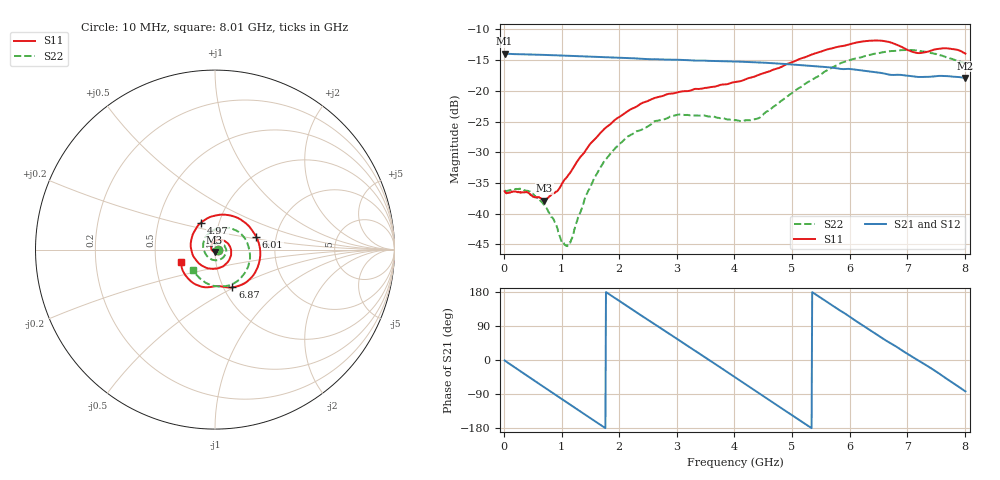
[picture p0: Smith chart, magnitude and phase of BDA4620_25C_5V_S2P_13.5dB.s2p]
!Agilent Technologies,E5071B,MY42404982,A.09.10
!Date: Wed May 06 09:01:02 2026
!Data & Calibration Information:
!Freq	S11:SOLT2(ON)	S21:SOLT2(ON)	S12:SOLT2(ON)	S22:SOLT2(ON)
# Hz S RI R 50
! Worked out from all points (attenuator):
!   801 points, 10 MHz to 8.01 GHz, reference 50 ohm
!   highest |S21| = -13.93 dB at 10 MHz (marker M1); lowest = -17.9 dB at 8.01 GHz (marker M2)
!   lowest |S11| = -37.9 dB at 700 MHz (marker M3), VSWR 1.03, Z = 49.7 - j1.24 ohm
!   |S11| at or under -10 dB: start of sweep to end of sweep
!   |S22| runs from -45.3 to -13.3 dB; largest |S21 - S12| = 0.0009
!   S11 on the Smith chart (normalised r, x): 10 MHz: 1.03, -0.00; 4.97 GHz: 0.82, +0.25; 6.01 GHz: 1.57, +0.24; 6.87 GHz: 1.10, -0.49; 8.01 GHz: 0.68, -0.10
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1e7  0.0152 -0.00103  0.2011 -0.00428  0.2014 -0.00438  0.0154 -0.000666
4.4e8  0.00868 -0.0117  0.1385 -0.1413  0.1386 -0.1417  0.0135 -0.00702
7e8  -0.00256 -0.0125  0.06 -0.1868  0.0599 -0.1872  0.00726 -0.00918
1.08e9  -0.0195 0.00114  -0.0692 -0.1807  -0.0695 -0.181  -0.00435 -0.00332
1.16e9  -0.0208 0.00685  -0.0938 -0.1686  -0.0942 -0.1687  -0.00598 -0.000482
1.35e9  -0.0211 0.0211  -0.1433 -0.1271  -0.1434 -0.1272  -0.00816 0.00748
1.59e9  -0.0112 0.0395  -0.1809 -0.0565  -0.1812 -0.0566  -0.00604 0.0194
1.9e9  0.0164 0.0542  -0.1816 0.0451  -0.1818 0.0452  0.00652 0.0323
2.31e9  0.0618 0.0422  -0.1046 0.1508  -0.1048 0.151  0.0331 0.0333
2.68e9  0.0893 -0.000602  0.00629 0.1806  0.00643 0.1809  0.0544 0.0177
3.39e9  0.0334 -0.0981  0.1687 0.0518  0.1691 0.0516  0.0459 -0.0429
4.01e9  -0.0879 -0.0786  0.1217 -0.1236  0.1218 -0.124  -0.0233 -0.0532
4.42e9  -0.1345 0.0105  0.00941 -0.17  0.00913 -0.1702  -0.0594 -0.00904
4.97e9  -0.0785 0.1499  -0.1307 -0.0997  -0.131 -0.0998  -0.0397 0.0852
5.35e9  0.0362 0.195  -0.1592 0.0025  -0.1594 0.0024  0.0303 0.1189
6.01e9  0.2292 0.0727  -0.0597 0.1383  -0.0598 0.1387  0.1692 0.0582
6.35e9  0.2474 -0.0661  0.0272 0.1411  0.0273 0.1414  0.1948 -0.0243
6.68e9  0.1679 -0.1859  0.0928 0.0992  0.093 0.0995  0.1765 -0.1129
6.87e9  0.0971 -0.2102  0.1178 0.0663  0.1181 0.0663  0.1464 -0.1558
7.19e9  0.0155 -0.2023  0.1298 -0.00252  0.1301 -0.00237  0.0645 -0.2032
7.56e9  -0.0852 -0.203  0.1065 -0.0784  0.1069 -0.0786  -0.0368 -0.1919
8.01e9  -0.1886 -0.0698  0.016 -0.1264  0.0163 -0.1268  -0.1225 -0.1134
